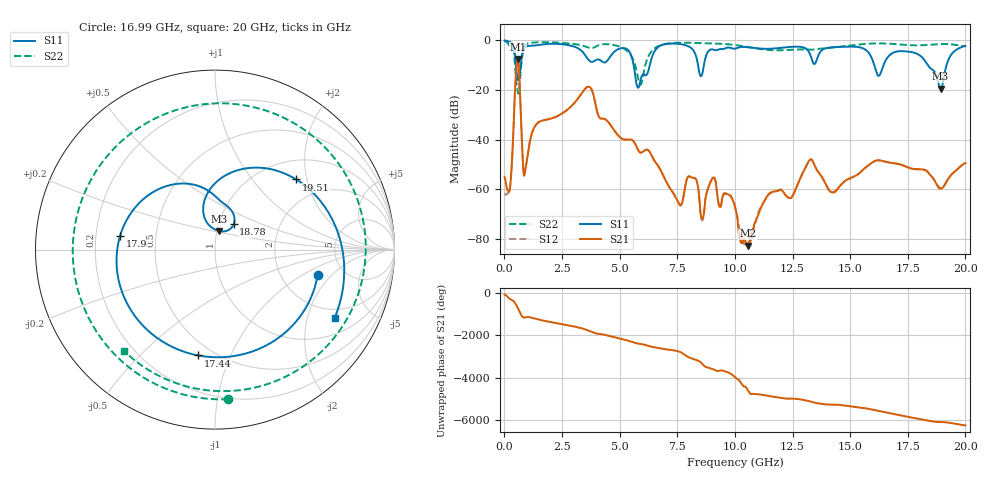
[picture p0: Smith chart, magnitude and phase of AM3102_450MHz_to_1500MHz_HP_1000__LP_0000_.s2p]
!Agilent Technologies,E8364B,MY43040894,A.07.50.67
!Agilent E8364B: A.07.50.67
!Date: Thursday, January 11, 2018 05:56:09
!Correction: S11(Full 2 Port(1,2))
!S21(Full 2 Port(1,2))
!S12(Full 2 Port(1,2))
!S22(Full 2 Port(1,2))
!S2P File: Measurements: S11, S21, S12, S22:
# Hz S  dB  R 50
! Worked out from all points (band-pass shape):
!   1601 points, 10 MHz to 20 GHz, reference 50 ohm
!   highest |S21| = -7.53 dB at 584.7 MHz (marker M1); lowest = -82.8 dB at 10.55 GHz (marker M2)
!   |S21| within 3 dB of the highest: 527.7 MHz to 628.2 MHz (100.6 MHz wide, 17.4 % of centre)
!   lowest |S11| = -19.5 dB at 18.93 GHz (marker M3), VSWR 1.24, Z = 51.4 + j10.8 ohm
!   |S11| at or under -10 dB: 5.607 GHz to 6.309 GHz (702 MHz wide, 11.8 % of centre); 16.05 GHz to 16.45 GHz (401.1 MHz wide, 2.47 % of centre); 18.37 GHz to 19.18 GHz (811.6 MHz wide, 4.32 % of centre)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
!   |S22| runs from -21.5 to -0.3 dB; largest |S21 - S12| = 0.0014
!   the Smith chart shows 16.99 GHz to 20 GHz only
!   S11 on the Smith chart (normalised r, x): 16.99 GHz: 3.21, -1.39; 17.44 GHz: 0.42, -0.76; 17.9 GHz: 0.30, +0.06; 18.78 GHz: 1.18, +0.34; 19.51 GHz: 1.42, +1.73; 20 GHz: 1.59, -2.97
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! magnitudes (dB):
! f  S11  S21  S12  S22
! 10 MHz  -0.1  -55.1  -61.9  -0.3
! 247.4 MHz  -0.7  -59.3  -59.2  -2.6
! 584.7 MHz  -15.7  -7.5  -7.5  -20.9
! 897.1 MHz  -2.8  -52.7  -52.6  -1.9
! 1.372 GHz  -2.0  -34.0  -34.0  -0.8
! 3.346 GHz  -4.2  -21.5  -21.5  -2.0
! 5.295 GHz  -3.4  -40.0  -40.0  -4.0
! 5.807 GHz  -19.1  -44.3  -44.3  -15.6
! 6.682 GHz  -2.7  -50.7  -50.7  -2.3
! 8.581 GHz  -13.7  -71.8  -72.6  -1.1
! 10.01 GHz  -3.4  -67.2  -66.8  -1.9
! 10.55 GHz  -2.8  -82.8  -82.1  -2.7
! 13.34 GHz  -7.8  -48.2  -48.2  -3.8
! 14.24 GHz  -2.8  -61.3  -61.2  -2.9
! 16.68 GHz  -6.3  -49.2  -49.2  -1.3
! 16.99 GHz  -4.6  -49.6  -49.7  -1.5
! 17.44 GHz  -4.5  -50.9  -51.0  -1.9
! 17.9 GHz  -5.4  -51.9  -52.0  -2.0
! 18.78 GHz  -15.1  -58.5  -58.2  -1.6
! 18.93 GHz  -19.5  -59.8  -59.5  -1.5
! 19.51 GHz  -4.5  -53.1  -53.1  -1.8
! 20 GHz  -2.3  -49.5  -49.4  -2.4
